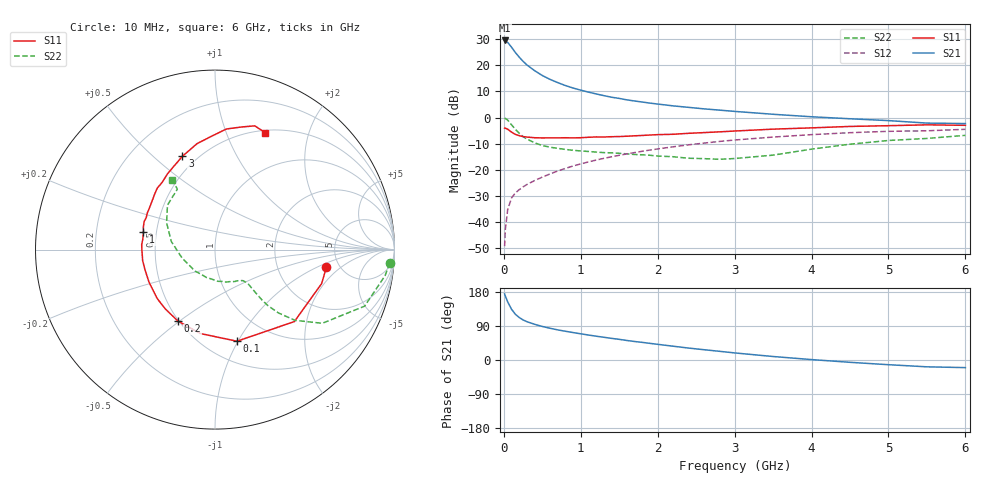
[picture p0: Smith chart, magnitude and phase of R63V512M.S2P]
! SIEMENS Small Signal Semiconductors
! BFR193
! Si NPN RF Bipolar Junction Transistor in SOT23
! VCE = 3.5 V  IC = 12 mA
! Common Emitter S-Parameters:  May  1996
# GHz  S  MA  R  50
!  f  S11  S21  S12  S22
! GHz  MAG  ANG  MAG  ANG  MAG  ANG  MAG  ANG
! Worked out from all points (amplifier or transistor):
!   36 points, 10 MHz to 6 GHz, reference 50 ohm
!   highest |S21| = 29.6 dB at 10 MHz (marker M1)
!   |S21| within 3 dB of that: start of sweep to 110.1 MHz
!   unconditionally stable (mu >= 1): 691.9 MHz to 1.911 GHz
!   at 250 MHz: K = 0.70, MSG = 24.1 dB, |S12| = -26.6 dB
!   at 1.4 GHz: K = 1.04, MAG = 10.3 dB, |S12| = -15.1 dB
!   at 6 GHz: K = 0.95, MSG = 1.1 dB, |S12| = -4.5 dB
!   S11 on the Smith chart (normalised r, x): 10 MHz: 3.93, -1.29; 100 MHz: 0.70, -0.99; 200 MHz: 0.49, -0.49; 1 GHz: 0.42, +0.10; 3 GHz: 0.42, +0.62; 6 GHz: 0.53, +1.38
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0.01  0.6285 -9.1  30.14 174.3  0.0034 87.2  0.9769 -4.4
0.02  0.6235 -17.7  29.62 168.6  0.0072 83.1  0.9587 -8.7
0.05  0.5969 -42.2  27.63 153.4  0.0171 72.9  0.8913 -20.7
0.1  0.525 -76.5  22.38 133.9  0.0286 63.4  0.725 -34.5
0.15  0.4746 -100.0  17.67 120.7  0.0358 58.4  0.5945 -41.5
0.2  0.4486 -117.4  14.43 112.1  0.0413 57.4  0.4984 -45.0
0.25  0.431 -130.1  11.98 105.7  0.0466 57.7  0.43 -46.6
0.3  0.422 -139.6  10.23 101.1  0.0519 58.6  0.3868 -47.0
0.4  0.4099 -153.8  7.932 94.2  0.0617 60.6  0.3275 -46.7
0.5  0.4059 -163.8  6.408 88.5  0.0719 62.6  0.2902 -46.3
0.6  0.4077 -171.3  5.404 83.8  0.0828 63.6  0.2696 -46.0
0.8  0.4094 176.1  4.113 75.9  0.1055 64.3  0.2443 -47.0
1  0.4103 166.4  3.35 69.1  0.1289 64.6  0.2285 -49.0
1.1  0.418 162.8  3.074 65.9  0.1409 64.1  0.2231 -51.3
1.3  0.4227 155.0  2.631 60.0  0.1647 62.8  0.2122 -55.0
1.6  0.4382 144.5  2.182 51.5  0.2004 60.4  0.2006 -63.2
2.2  0.4772 127.9  1.674 36.4  0.2741 54.0  0.1769 -85.4
3  0.5509 109.2  1.312 18.7  0.3705 42.9  0.1634 -133.0
3.5  0.5988 99.6  1.155 9.2  0.422 35.3  0.1899 -166.1
4.5  0.6748 84.6  0.947 -6.1  0.5119 20.5  0.308 151.1
5.5  0.7242 72.2  0.782 -18.0  0.5568 5.4  0.3969 121.9
6  0.7091 66.7  0.766 -20.1  0.5942 0.9  0.4552 121.5
